(* 	
	Program Name: 	ACS_DRIVE_INPUT_SCAN
	Purpose:		Copy Drive Inputs into shadow memory for user access
*)
PROGRAM ACS_DRIVE_INPUT_SCAN
VAR_IN_OUT
	Axis:ACS_DRIVE_TYPE;
END_VAR

//Run Input Scan Sub Routines
ACS_READ_AXIS_BITS( Axis:= Axis);
ACS_READ_AXIS_VARIABLES(Axis:= Axis);

END_PROGRAM
